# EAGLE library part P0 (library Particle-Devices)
Particle P0 module (WiFi without antenna)
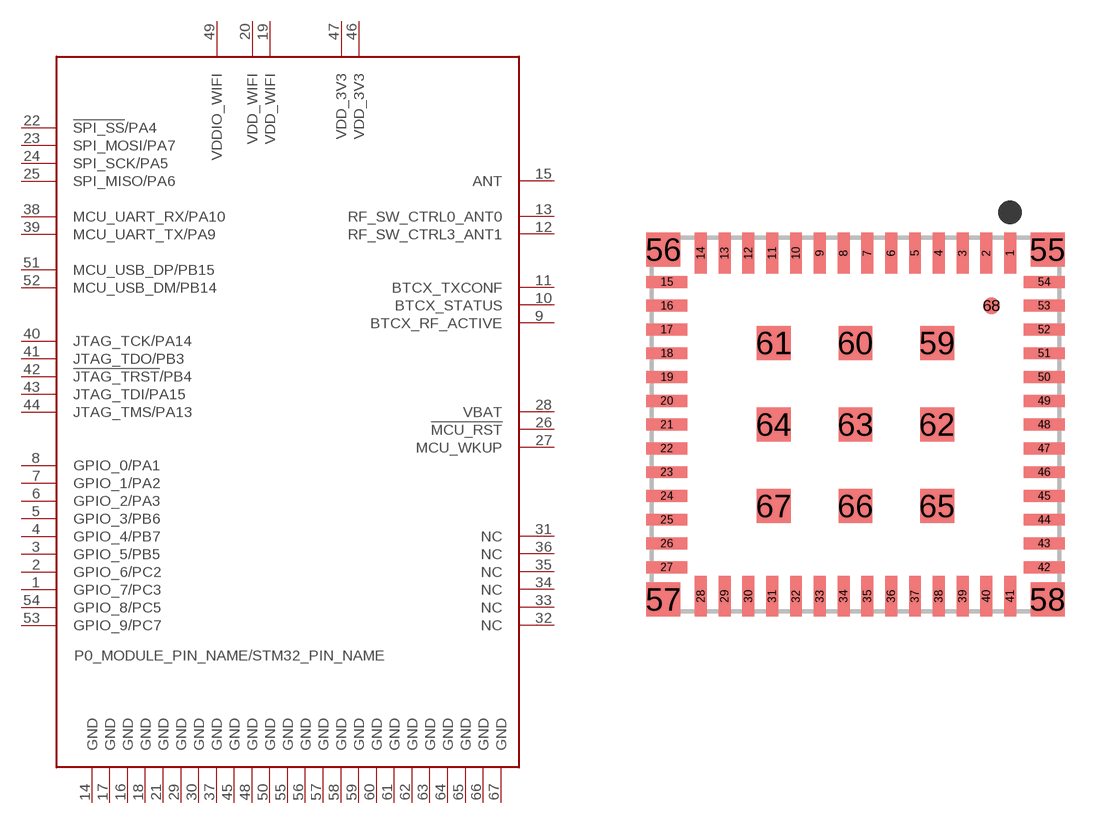
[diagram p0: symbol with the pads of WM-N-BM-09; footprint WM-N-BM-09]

Designator prefix U

## P0  [WM-N-BM-09]
1  GPIO_7/PC3
2  GPIO_6/PC2
3  GPIO_5/PB5
4  GPIO_4/PB7
5  GPIO_3/PB6
6  GPIO_2/PA3
7  GPIO_1/PA2
8  GPIO_0/PA1
9  BTCX_RF_ACTIVE
10  BTCX_STATUS
11  BTCX_TXCONF
12  RF_SW_CTRL3_ANT1
13  RF_SW_CTRL0_ANT0
14  GND
15  ANT
16  GND
17  GND
18  GND
19  VDD_WIFI
20  VDD_WIFI
21  GND
22  !SPI_SS!/PA4
23  SPI_MOSI/PA7
24  SPI_SCK/PA5
25  SPI_MISO/PA6
26  !MCU_RST
27  MCU_WKUP
28  VBAT
29  GND
30  GND
31  NC
32  NC
33  NC
34  NC
35  NC
36  NC
37  GND
38  MCU_UART_RX/PA10
39  MCU_UART_TX/PA9
40  JTAG_TCK/PA14
41  JTAG_TDO/PB3
42  !JTAG_TRST!/PB4
43  JTAG_TDI/PA15
44  JTAG_TMS/PA13
45  GND
46  VDD_3V3
47  VDD_3V3
48  GND
49  VDDIO_WIFI
50  GND
51  MCU_USB_DP/PB15
52  MCU_USB_DM/PB14
53  GPIO_9/PC7
54  GPIO_8/PC5
55  GND
56  GND
57  GND
58  GND
59  GND
60  GND
61  GND
62  GND
63  GND
64  GND
65  GND
66  GND
67  GND

## Footprint WM-N-BM-09 (pad centres in mm)
WM-N-BM-09
smd 0.35 x 1.2: 1 4.55,5.05; 2 3.85,5.05; 3 3.15,5.05; 4 2.45,5.05; 5 1.75,5.05; 6 1.05,5.05; 7 0.35,5.05; 8 -0.35,5.05; 9 -1.05,5.05; 10 -1.75,5.05; 11 -2.45,5.05; 12 -3.15,5.05; 13 -3.85,5.05; 14 -4.55,5.05; 28 -4.55,-5.05; 29 -3.85,-5.05; 30 -3.15,-5.05; 31 -2.45,-5.05; 32 -1.75,-5.05; 33 -1.05,-5.05; 34 -0.35,-5.05; 35 0.35,-5.05; 36 1.05,-5.05; 37 1.75,-5.05; 38 2.45,-5.05; 39 3.15,-5.05; 40 3.85,-5.05; 41 4.55,-5.05
smd 1.2 x 0.35: 15 -5.55,4.2; 16 -5.55,3.5; 17 -5.55,2.8; 18 -5.55,2.1; 19 -5.55,1.4; 20 -5.55,0.7; 21 -5.55,0; 22 -5.55,-0.7; 23 -5.55,-1.4; 24 -5.55,-2.1; 25 -5.55,-2.8; 26 -5.55,-3.5; 27 -5.55,-4.2; 42 5.55,-4.2; 43 5.55,-3.5; 44 5.55,-2.8; 45 5.55,-2.1; 46 5.55,-1.4; 47 5.55,-0.7; 48 5.55,0; 49 5.55,0.7; 50 5.55,1.4; 51 5.55,2.1; 52 5.55,2.8; 53 5.55,3.5; 54 5.55,4.2
smd 1 x 1: 55 5.65,5.15; 56 -5.65,5.15; 57 -5.65,-5.15; 58 5.65,-5.15; 59 2.4,2.4; 60 0,2.4; 61 -2.4,2.4; 62 2.4,0; 63 0,0; 64 -2.4,0; 65 2.4,-2.4; 66 0,-2.4; 67 -2.4,-2.4
smd 0.5 x 0.5: 68 4,3.5

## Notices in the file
Licensing: Designed by Particle.
